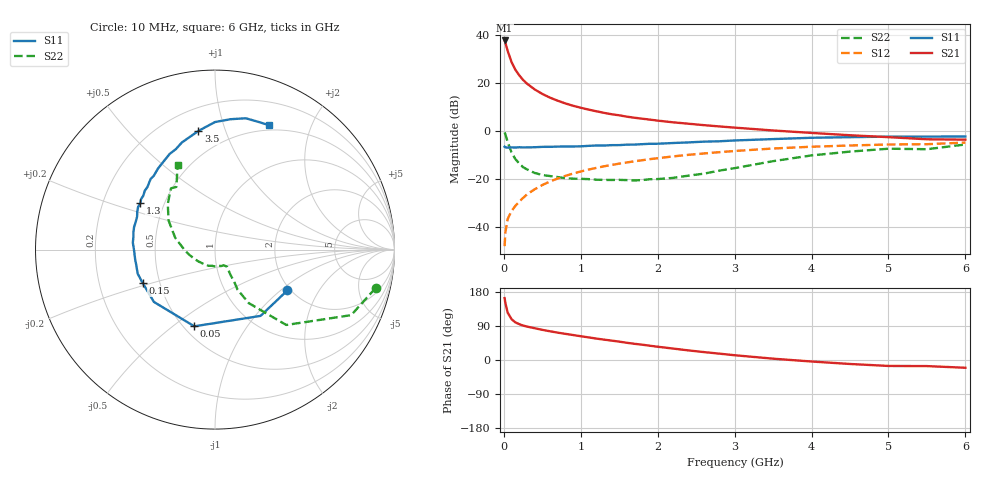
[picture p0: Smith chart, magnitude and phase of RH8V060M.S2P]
! SIEMENS Small Signal Semiconductors
! BFR106
! Si NPN RF Bipolar Junction Transistor in SOT23
! VCE = 8 V  IC = 60 mA
! Common Emitter S-Parameters:  August  1996
# GHz  S  MA  R  50
!  f  S11  S21  S12  S22
! GHz  MAG  ANG  MAG  ANG  MAG  ANG  MAG  ANG
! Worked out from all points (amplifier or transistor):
!   36 points, 10 MHz to 6 GHz, reference 50 ohm
!   highest |S21| = 37.6 dB at 10 MHz (marker M1)
!   |S21| within 3 dB of that: start of sweep to 38 MHz
!   unconditionally stable (mu >= 1): 236.8 MHz to 2.299 GHz
!   at 250 MHz: K = 1.01, MAG = 23.9 dB, |S12| = -28.0 dB
!   at 1.4 GHz: K = 1.06, MAG = 9.1 dB, |S12| = -14.3 dB
!   at 6 GHz: K = 0.98, MSG = 0.6 dB, |S12| = -5.0 dB
!   S11 on the Smith chart (normalised r, x): 10 MHz: 1.92, -1.12; 50 MHz: 0.56, -0.60; 150 MHz: 0.40, -0.18; 1.3 GHz: 0.37, +0.25; 3.5 GHz: 0.34, +0.81; 6 GHz: 0.44, +1.43
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0.01  0.4627 -29.5  76.08 163.3  0.0039 79.9  0.9198 -13.5
0.02  0.4482 -55.5  68.59 150.2  0.0076 70.3  0.842 -25.7
0.05  0.4427 -105.1  45.84 124.9  0.0144 60.0  0.5779 -46.6
0.1  0.4481 -139.4  27.03 107.8  0.0211 62.1  0.3518 -57.8
0.15  0.4441 -155.4  18.65 99.3  0.027 64.2  0.2553 -60.6
0.2  0.4512 -162.8  14.27 94.6  0.0331 67.9  0.2066 -59.1
0.25  0.447 -169.1  11.46 90.9  0.0396 69.5  0.1732 -58.7
0.3  0.4481 -172.8  9.584 88.3  0.0467 70.3  0.1561 -58.1
0.4  0.4511 -179.5  7.263 83.9  0.0598 72.0  0.1313 -56.1
0.5  0.4594 175.2  5.828 79.6  0.0734 71.9  0.1189 -54.8
0.6  0.4602 171.0  4.884 75.8  0.0873 71.5  0.113 -55.8
0.7  0.4652 167.6  4.218 72.2  0.1005 71.1  0.1077 -57.9
0.9  0.4678 160.9  3.306 65.9  0.1276 68.8  0.0997 -61.2
1.1  0.4821 154.0  2.753 59.7  0.1542 66.6  0.0976 -69.7
1.3  0.4891 148.1  2.356 53.8  0.1802 64.0  0.0939 -77.0
1.7  0.5128 137.2  1.858 42.7  0.23 58.7  0.0917 -99.3
2.2  0.5526 125.0  1.493 30.2  0.2904 51.6  0.1035 -131.3
2.8  0.6006 111.3  1.226 16.8  0.3558 42.8  0.1467 -168.9
3.5  0.6675 98.0  1.009 3.5  0.4245 32.7  0.2312 163.5
4.5  0.7316 83.2  0.803 -10.5  0.4904 18.0  0.3658 136.0
5.5  0.7519 70.7  0.661 -16.1  0.5221 8.0  0.4104 121.6
6  0.7558 66.4  0.65 -20.5  0.5649 1.0  0.5147 113.9
